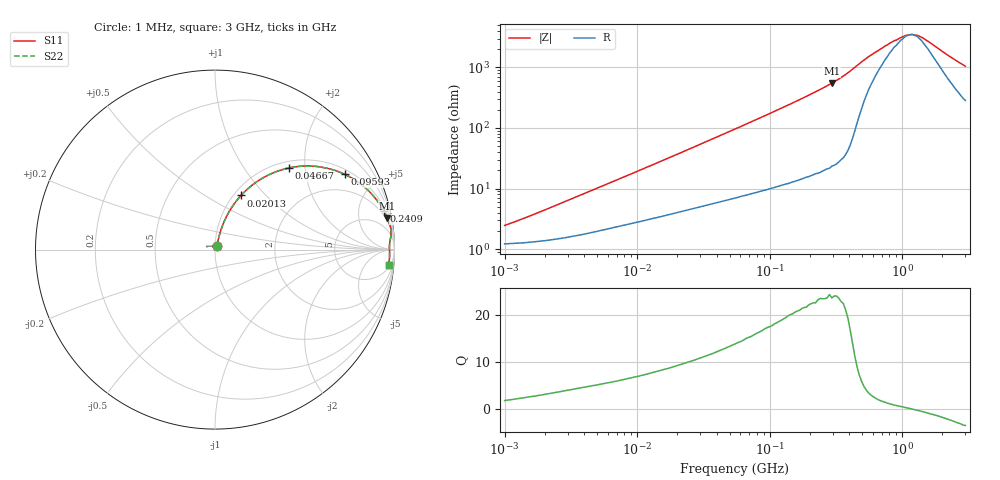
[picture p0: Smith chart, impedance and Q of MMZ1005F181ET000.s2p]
! S-parameter Generated by TDK Corporation
! Copyright(C) 2018 TDK Corporation.
! All Rights Reserved.
! TDK P/N: MMZ1005F181ET000 (Chip Bead)
! Property: |Z|=180¶ at 100MHz
! Size(LxWxT): 1x0.5x0.5mm, 0.039x0.02x0.02inches
! Model Type: s2p (Touchstone File Format Version 1.0)
! Frequency: DC=Yes Start=1MHz Stop=3000MHz 202points Log-sweep
! Model Generated on Aug. 6, 2018
! Port Assignments:
!  1 ---@@@--- 2
! Applicable Conditions:
!  Temperature = 25 degC
!  DC Bias Current = 0 A
!  Small Signal Operation
! Terms and conditions regarding TDK Simulation Models
! (1)This simulation model is being provided solely for informational purposes. Please refer to the specifications of the products in terms of detailed characteristics of such products.
! (2)In no event shall TDK Corporation of any of its subsidiaries be liable for any loss or damage arising, directly or indirectly,
!  From any information contained in this simulation model, including, but not limited to loss or damages arising from any inaccuracies, omissions or errors in connection with such information.
! (3)Any and all copyrights on this simulation model are owned by TDK Corporation.
!  Duplication or redistribution of this simulation model without prior written permission from TDK Corporation is prohibited.
! (4)This simulation model is subject to any modification or change without any prior notice.
! (5)Neither TDK Corporation nor any of its subsidiaries shall make any warranty, express or implied,
!  Including but not limited to the correctness, implied warranties of merchantability and fitness for a particular purpose with respect to this simulation models.
! (6)The use of this simulation model shall be deemed to have consented to the terms and conditions hereof.
# Hz S MA R 50
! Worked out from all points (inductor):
!   201 points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, 1 MHz to 3 GHz, reference 50 ohm
!   read as one part in series: L = 331 nH near 1.975 MHz
!   highest Q = 23.9 at 294.3 MHz (marker M1), where L = 297 nH
!   self-resonance near 1.168 GHz
!   S11 on the Smith chart (normalised r, x): 1 MHz: 1.02, +0.04; 20.13 MHz: 1.08, +0.73; 46.67 MHz: 1.13, +1.64; 95.93 MHz: 1.19, +3.32; 240.9 MHz: 1.37, +8.67; 3 GHz: 7, -20
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1000000  0.02425 59.1  0.9878 -1.2  0.9878 -1.2  0.02425 59.1
3900413  0.07928 73.1  0.9799 -4.4  0.9799 -4.4  0.07928 73.1
7703107  0.1457 72.4  0.9661 -8.3  0.9661 -8.3  0.1457 72.4
1.461624e7  0.2557 68.2  0.9356 -14.7  0.9356 -14.7  0.2557 68.2
2.013356e7  0.3348 64.3  0.9067 -19.4  0.9067 -19.4  0.3348 64.3
3.127247e7  0.4711 56.8  0.8403 -28.0  0.8403 -28.0  0.4711 56.8
4.666789e7  0.6125 47.9  0.7445 -37.6  0.7445 -37.6  0.6125 47.9
5.477226e7  0.6688 44.0  0.6966 -41.8  0.6966 -41.8  0.6688 44.0
7.248696e7  0.7598 37.0  0.6026 -49.3  0.6026 -49.3  0.7598 37.0
9.593103e7  0.8356 30.1  0.503 -56.5  0.503 -56.5  0.8356 30.1
1.431579e8  0.912 21.5  0.367 -65.6  0.367 -65.6  0.912 21.5
2.136344e8  0.9565 14.6  0.2523 -72.8  0.2523 -72.8  0.9565 14.6
2.408952e8  0.9655 12.9  0.2226 -74.7  0.2226 -74.7  0.9655 12.9
2.942768e8  0.9766 10.2  0.1777 -77.3  0.1777 -77.3  0.9766 10.2
3.741707e8  0.9856 7.4  0.1288 -79.9  0.1288 -79.9  0.9856 7.4
4.951867e8  0.9834 4.5  0.07925 -75.7  0.07925 -75.7  0.9834 4.5
8.005644e8  0.9728 1.6  0.03906 -45.2  0.03906 -45.2  0.9728 1.6
1.059487e9  0.972 0.4  0.02886 -14.1  0.02886 -14.1  0.972 0.4
1.194682e9  0.9723 -0.1  0.02773 3.7  0.02773 3.7  0.9723 -0.1
1.294266e9  0.9727 -0.5  0.02852 16.3  0.02852 16.3  0.9727 -0.5
1.45942e9  0.973 -1.0  0.0325 33.2  0.0325 33.2  0.973 -1.0
3e9  0.9708 -5.1  0.09255 69.1  0.09255 69.1  0.9708 -5.1
